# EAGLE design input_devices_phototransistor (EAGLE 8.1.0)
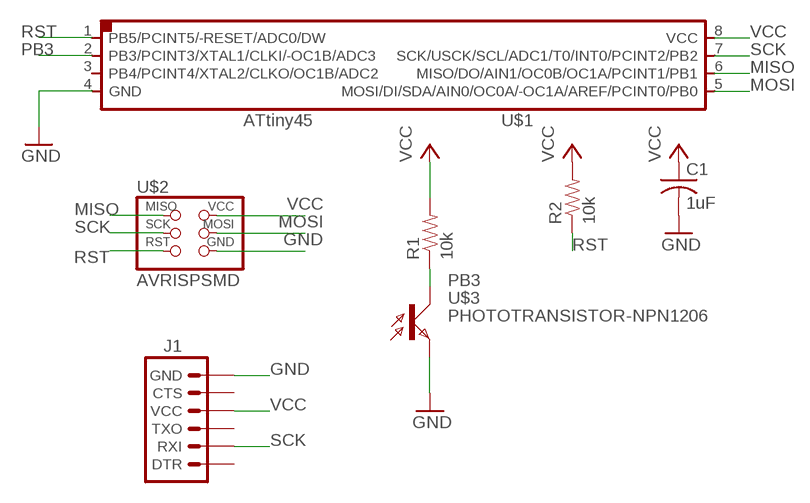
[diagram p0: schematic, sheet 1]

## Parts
C1  1uF  C-USC0805  [C0805]
J1  ARDUINO_SERIAL_PROGRAMSMD  [1X06-SMD]
R1  10k  RESISTOR1206  [1206]
R2  10k  RESISTOR1206  [1206]
U$1  ATTINY45SI  [SOIC8]
U$2  AVRISPSMD  [2X03SMD]
U$3  PHOTOTRANSISTOR-NPN1206  [OP1206]

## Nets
GND: C1.2 J1.6(GND) U$1.4(GND) U$2.6(GND) U$3.EMITTER(E)
MISO: U$1.6(MISO/DO/AIN1/OC0B/OC1A/PCINT1/PB1) U$2.1(MISO)
MOSI: U$1.5(MOSI/DI/SDA/AIN0/OC0A/-OC1A/AREF/PCINT0/PB0) U$2.4(MOSI)
PB3: R1.1 U$1.2(PB3/PCINT3/XTAL1/CLKI/-OC1B/ADC3) U$3.COLLECTOR(C)
RST: R2.1 U$1.1(PB5/PCINT5/-RESET/ADC0/DW) U$2.5(RST)
SCK: J1.2(RXI) U$1.7(SCK/USCK/SCL/ADC1/T0/INT0/PCINT2/PB2) U$2.3(SCK)
VCC: C1.1 J1.4(VCC) R1.2 R2.2 U$1.8(VCC) U$2.2(VCC)
Unconnected: J1.1(DTR) J1.3(TXO) J1.5(CTS) U$1.3(PB4/PCINT4/XTAL2/CLKO/OC1B/ADC2)

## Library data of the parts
C1 = rcl:C-US: CAPACITOR, American symbol
J1 = SparkFun-Connectors:ARDUINO_SERIAL_PROGRAM: FTDI connector footprints; PROD_ID: CONN-08971
R1 R2 = SparkFun-Passives:RESISTOR: Resistor
U$1 = fab:ATTINY45
U$2 = fab:AVRISP
U$3 = fab:PHOTOTRANSISTOR-NPN

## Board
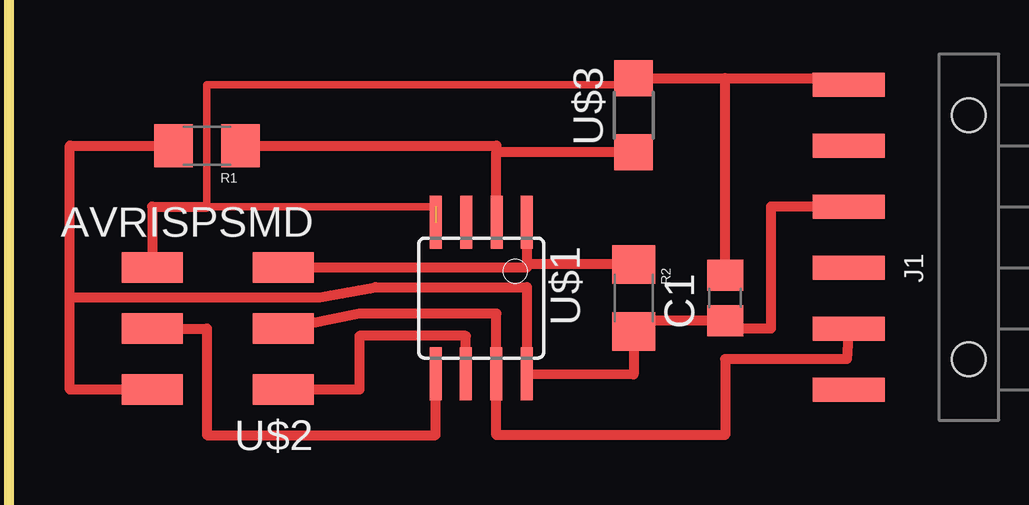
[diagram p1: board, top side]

No outline drawn. Coordinates in mm, seen from the top.
Copper layers (1*16): Top 0.035mm / dielectric 1.5mm / Bottom 0.035mm
Design rules "default *": minimum track width 10mil, minimum drill 24mil, track to track 16mil, track to pad 16mil, pad to pad 16mil, via to via 16mil, smd to smd 16mil, copper to edge 40mil, drill to drill 8mil, minimum pad ring 10mil, minimum via ring 8mil, stop-mask expansion 4mil, vias tented up to drill 0mil, thermal gap 10mil
Milling: 4 lines

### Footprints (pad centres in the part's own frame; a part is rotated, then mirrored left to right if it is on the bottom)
C0805 = smd 1.3 x 1.5: 1 -0.95,0; 2 0.95,0
1X06-SMD = smd 1 x 3: 1 -6.35,5; 2 -3.81,5; 3 -1.27,5; 4 1.27,5; 5 3.81,5; 6 6.35,5 | hole 1.4: -5.08,0; 5.08,0
1206 = smd 1.6 x 1.8: 1 -1.4,0; 2 1.4,0
SOIC8 = smd 0.5 x 2.2: 1 -1.905,-3.154; 2 -0.645,-3.154; 3 0.625,-3.154; 4 1.895,-3.154; 5 1.905,3.154; 6 0.635,3.154; 7 -0.635,3.154; 8 -1.905,3.154
2X03SMD = smd 2.54 x 1.27: 1 -2.54,2.54; 2 2.92,2.54; 3 -2.54,0; 4 2.92,0; 5 -2.54,-2.54; 6 2.92,-2.54
OP1206 = smd 1.5 x 1.6: COLLECTOR -1.55,0; EMITTER 1.55,0

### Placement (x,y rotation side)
C1  29.84,9.53 90 top
J1  40.01,12.06 90 top
R1  8.26,15.88 180 top
R2  26.04,9.53 270 top
U$1  19.68,9.53 180 top
U$2  8.89,8.26 180 top
U$3  26.04,17.14 90 top

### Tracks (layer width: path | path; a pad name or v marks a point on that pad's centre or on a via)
GND  (2 unrouted)
  Top 0.305: U$3.EMITTER 26.04,18.41 8.26,18.41 8.26,13.34 17.78,13.34
  Top 0.406: U$1.4 | U$3.EMITTER 29.84,18.7 | 29.84,18.7 35.01,18.7 J1.6 | C1.2 29.84,18.7 | 8.26,13.34 5.97,13.34 U$2.6
MISO
  Top 0.406: U$1.6 19.05,7.95 14.61,7.95 14.61,5.71 U$2.1
MOSI
  Top 0.406: U$2.4 8.26,8.26 8.26,3.81 17.78,3.81 U$1.5
PB3
  Top 0.406: 20.32,15.6 20.32,15.88 R1.1 | 20.32,15.6 20.32,13.34 20.33,13.34 U$1.2 | U$3.COLLECTOR 20.32,15.6
RST
  Top 0.406: R2.1 21.59,10.93 | 21.59,10.93 21.59,10.79 U$2.5 | U$1.1 21.59,10.93
SCK
  Top 0.406: U$2.3 14.61,8.89 20.32,8.89 U$1.7 20.32,3.81 29.84,3.81 29.84,6.99 34.92,6.99 J1.2
VCC
  Top 0.406: U$2.2 2.54,5.71 2.54,9.53 | J1.4 31.75,13.34 31.75,8.26 29.84,8.26 C1.1 26.04,8.57 R2.2 26.04,6.35 U$1.8 21.59,9.98 15.29,9.98 12.95,9.55 2.56,9.55 2.54,9.53 | 2.54,9.53 2.54,15.88 R1.2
